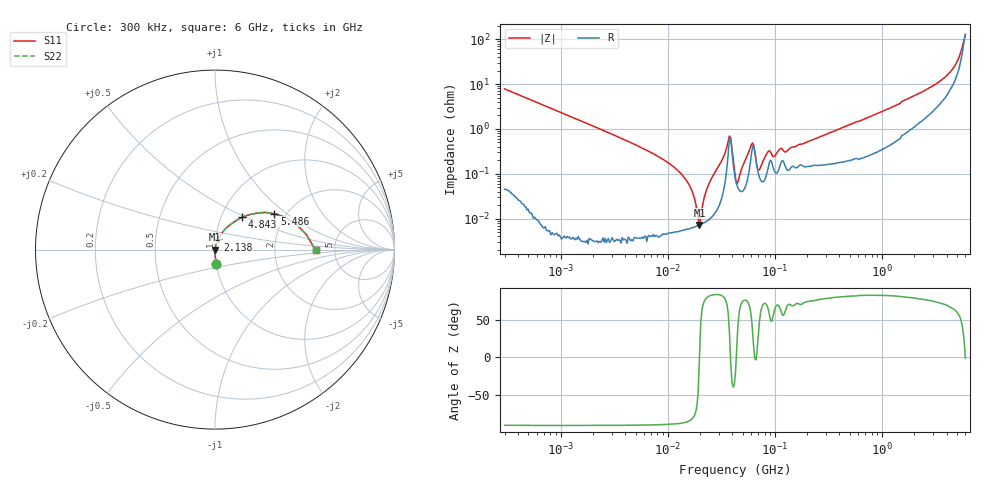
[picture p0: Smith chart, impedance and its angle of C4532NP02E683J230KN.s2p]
! S-Parameter Data Generated by TDK Corporation
! Copyright(C) 2024 TDK Corporation.
! All Rights Reserved.
! TDK P/N: C4532NP02E683J230KN (Multilayer Ceramic Chip Capacitor)
! Property: C=68nF
! Size(LxWxT): 4.5x3.2x2.3mm
! Model Type: s2p (Touchstone File Format Version 1.0)
! Frequency: DC=Yes Start=0.3MHz Stop=6000MHz 402points Log-sweep
! Model Generated on May 28, 2024
! Terms and conditions regarding TDK Simulation Models:
! 1)This simulation model is being provided solely for informational
!  purposes. Please refer to the specifications of the products in
!  terms of detailed characteristics of such products.
! 2)In no event shall TDK Corporation of any of its subsidiaries be
!  liable for any loss or damage arising, directly or indirectly,
!  from any information contained in this simulation model, including,
!  but not limited to loss or damages arising from any inaccuracies,
!  omissions or errors in connection with such information.
! 3)Any and all copyrights on this simulation model are owned by
!  TDK Corporation.  Duplication or redistribution of this simulation
!  model without prior written permission from TDK Corporation
!  is prohibited.
! 4)This simulation model is subject to any modification or change
!  without any prior notice.
! 5)Neither TDK Corporation nor any of its subsidiaries shall make any
!  warranty, express or implied, including but not limited to the
!  correctness, implied warranties of merchantability and fitness for
!  a particular purpose with respect to this simulation models.
! 6)The use of this simulation model shall be deemed to have consented
!  to the terms and conditions hereof.
! Port Assignments:
!  1 ---| |--- 2
! Applicable Conditions:
!  Temperature = 25 degC
!  DC Bias Voltage = 0 V
!  Small Signal Operation
# Hz S MA R 50
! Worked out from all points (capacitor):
!   401 points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, 300 kHz to 6 GHz, reference 50 ohm
!   read as one part in series: C = 67.6 nF near 317.3 kHz
!   lowest |Z| = 7.21 mohm at 19.77 MHz (marker M1)
!   series resonance near 19.75 MHz, so ESL is about 960 pH
!   S11 on the Smith chart (normalised r, x): 300 kHz: 1.00, -0.16; 2.138 GHz: 1.03, +0.12; 4.843 GHz: 1.25, +0.48; 5.486 GHz: 1.74, +0.82; 6 GHz: 3.56, -0.05
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300000  0.07813 -85.2  0.9965 4.5  0.9965 4.5  0.07813 -85.2
1586297  0.01475 -89.0  0.9999 0.8  0.9999 0.8  0.01475 -89.0
8158352  0.002422 -88.9  1 0.1  1 0.1  0.002422 -88.9
1.472706e7  0.0007459 -85.6  0.9999 0.0  0.9999 0.0  0.0007459 -85.6
1.673422e7  0.0004282 -81.6  0.9999 0.0  0.9999 0.0  0.0004282 -81.6
1.976502e7  7.208e-05 1.7  0.9999 -0.0  0.9999 -0.0  7.208e-05 1.7
2.364199e7  0.0005199 79.8  0.9999 -0.0  0.9999 -0.0  0.0005199 79.8
3.261876e7  0.0022 80.7  0.9996 -0.1  0.9996 -0.1  0.0022 80.7
3.656965e7  0.005161 59.6  0.9974 -0.3  0.9974 -0.3  0.005161 59.6
3.867823e7  0.006251 -7.8  0.9938 0.0  0.9938 0.0  0.006251 -7.8
4.28954e7  0.0007955 -20.0  0.9993 0.0  0.9993 0.0  0.0007955 -20.0
4.605827e7  0.0007839 55.4  0.9996 -0.0  0.9996 -0.0  0.0007839 55.4
6.063722e7  0.004546 49.7  0.9971 -0.2  0.9971 -0.2  0.004546 49.7
7.161949e7  0.001227 46.5  0.9992 -0.1  0.9992 -0.1  0.001227 46.5
8.767476e7  0.003238 60.4  0.9984 -0.2  0.9984 -0.2  0.003238 60.4
9.881314e7  0.002433 61.8  0.9989 -0.1  0.9989 -0.1  0.002433 61.8
2.249926e8  0.005766 74.4  0.9985 -0.3  0.9985 -0.3  0.005766 74.4
1.174439e9  0.02882 79.8  0.9953 -1.6  0.9953 -1.6  0.02882 79.8
2.137749e9  0.05871 74.4  0.9858 -3.3  0.9858 -3.3  0.05871 74.4
4.843348e9  0.2354 50.0  0.8676 -12.0  0.8676 -12.0  0.2354 50.0
5.485933e9  0.3866 31.2  0.6987 -16.7  0.6987 -16.7  0.3866 31.2
6e9  0.5616 -0.5  0.4384 0.6  0.4384 0.6  0.5616 -0.5
